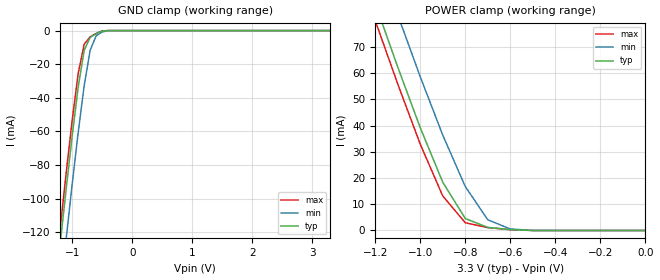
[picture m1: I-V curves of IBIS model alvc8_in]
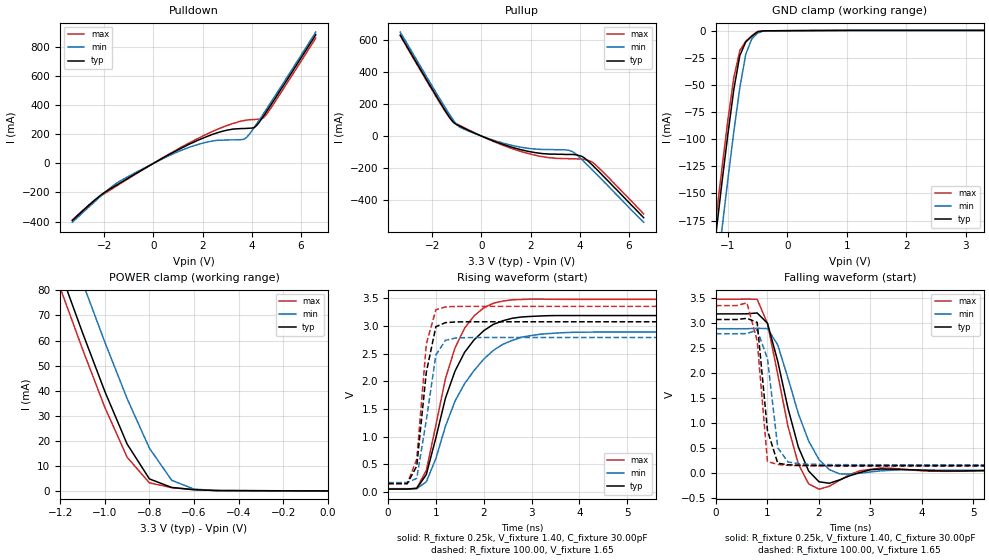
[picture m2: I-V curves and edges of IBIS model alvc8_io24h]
| IBIS file 32245ah.ibs created by s2ibis2 version 1.1
| North Carolina State University Electronics Research Laboratory  1995
[IBIS ver]   2.1
[File name]   32245ah.ibs
[File Rev]   1.0
[Date]   03/01/99
[Source]   Integrated Device Technology, Inc.
[Notes]   1.Temperatures: typ=25C, min=100C, max=0C 2.RRmp rates based
   on 50 ohm load.
[Disclaimer] Integrated Device Technology, Inc. ("IDT") hereby grants the
   user of this IBIS model a non-exclusive, nontransferable
   license to use this IBIS model under the following terms. The
   user is granted this license only to use the IBIS model and is
   not granted rights to sell, copy (except as needed to run the
   IBIS model), rent, lease or sub-license the IBIS model in
   whole or in part, or in modified form to anyone. The User may
   modify the IBIS model to suit its specific applications, but
   rights to derivative works and such modifications shall belong
   to IDT. This IBIS model is provided on an AS IS" basis and IDT
   makes absolutely no warranty with respect to the information
   contained herein. IDT DISCLAIMS AND CUSTOMER WAIVES ALL
   WARRANTIES, EXPRESS AND IMPLIED, INCLUDING WARRANTIES OF
   MERCHANTABILITY AND FITNESS FOR A PARTICULAR PURPOSE. THE
   ENTIRE RISK AS TO QUALITY AND PERFORMANCE IS WITH THE USER
   ACCORDINGLY, IN NO EVENT SHALL IDT BE LIABLE FOR ANY DIRECT OR
   INDIRECT DAMAGES, WHETHER IN CONTRACT OR TORT, INCLUDING ANY
   LOST PROFITS OR OTHER INCIDENTAL, CONSEQUENTIAL, EXEMPLARY, OR
   PUNITIVE DAMAGES ARISING OUT OF THE USE OR APPLICATION OF THE
   IBIS model. Further, IDT reserves the right to make changes
   without notice to any product herein to improve reliability,
   function, or design. IDT does not convey any license under
   patent rights or any other intellectual property rights,
   including those of third parties. IDT is not obligated to
   provide maintenance or support for the licensed IBIS model.
[Copyright]   Copyright 1997, Integrated Device Technology, Inc. all rights
   reserved
|   Component ALVCH32245
[Component]   ALVCH32245
[Manufacturer]   Integrated Device Technology
[Package]
| BF96
| variable   typ   min   max
R_pkg   144.3m   NA   NA
L_pkg   4.10nH   NA   NA
C_pkg   0.36pF   NA   NA
[Pin]  signal_name   model_name   R_pin   L_pin   C_pin
A1   1B2   alvc8_io24h
A2   1B1   alvc8_io24h
A3   1DIR   alvc8_in
A4   1OEB   alvc8_in
A5   1A1   alvc8_io24h
A6   1A2   alvc8_io24h
B1   1B4   alvc8_io24h
B2   1B3   alvc8_io24h
B3   GND   GND
B4   GND   GND
B5   1A3   alvc8_io24h
B6   1A4   alvc8_io24h
C1   1B6   alvc8_io24h
C2   1B5   alvc8_io24h
C3   VCC   POWER
C4   VCC   POWER
C5   1A5   alvc8_io24h
C6   1A6   alvc8_io24h
D1   1B8   alvc8_io24h
D2   1B7   alvc8_io24h
D3   GND   GND
D4   GND   GND
D5   1A7   alvc8_io24h
D6   1A8   alvc8_io24h
E1   2B2   alvc8_io24h
E2   2B1   alvc8_io24h
E3   GND   GND
E4   GND   GND
E5   2A1   alvc8_io24h
E6   2A2   alvc8_io24h
F1   2B4   alvc8_io24h
F2   2B3   alvc8_io24h
F3   VCC   POWER
F4   VCC   POWER
F5   2A3   alvc8_io24h
F6   2A4   alvc8_io24h
G1   2B6   alvc8_io24h
G2   2B5   alvc8_io24h
G3   GND   GND
G4   GND   GND
G5   2A5   alvc8_io24h
G6   2A6   alvc8_io24h
H1   2B7   alvc8_io24h
H2   2B8   alvc8_io24h
H3   2DIR   alvc8_in
H4   2OEB   alvc8_in
H5   2A8   alvc8_io24h
H6   2A7   alvc8_io24h
J1   3B2   alvc8_io24h
J2   3B1   alvc8_io24h
J3   3DIR   alvc8_in
J4   3OEB   alvc8_in
J5   3A1   alvc8_io24h
J6   3A2   alvc8_io24h
K1   3B4   alvc8_io24h
K2   3B3   alvc8_io24h
K3   GND   GND
K4   GND   GND
K5   3A3   alvc8_io24h
K6   3A4   alvc8_io24h
L1   3B6   alvc8_io24h
L2   3B5   alvc8_io24h
L3   VCC   POWER
L4   VCC   POWER
L5   3A5   alvc8_io24h
L6   3A6   alvc8_io24h
M1   3B8   alvc8_io24h
M2   3B7   alvc8_io24h
M3   GND   GND
M4   GND   GND
M5   3A7   alvc8_io24h
M6   3A8   alvc8_io24h
N1   4B2   alvc8_io24h
N2   4B1   alvc8_io24h
N3   GND   GND
N4   GND   GND
N5   4A1   alvc8_io24h
N6   4A2   alvc8_io24h
P1   4B4   alvc8_io24h
P2   4B3   alvc8_io24h
P3   VCC   POWER
P4   VCC   POWER
P5   4A3   alvc8_io24h
P6   4A4   alvc8_io24h
R1   4B6   alvc8_io24h
R2   4B5   alvc8_io24h
R3   GND   GND
R4   GND   GND
R5   4A5   alvc8_io24h
R6   4A6   alvc8_io24h
T1   4B7   alvc8_io24h
T2   4B8   alvc8_io24h
T3   4DIR   alvc8_in
T4   4OEB   alvc8_in
T5   4A8   alvc8_io24h
T6   4A7   alvc8_io24h
| Models and submodels in the file (2): alvc8_in (Input), alvc8_io24h (I/O)
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| in   in   dummy_model
| oe   oe   dummy_model
|   Model alvc8_in
[Model]   alvc8_in
Model_type   Input
Vinl =  0.800V
Vinh =  2.000V
C_comp   3.00pF   NA   NA
[Temperature Range]   25.00   100.00   0.000
[Voltage Range]   3.30V   3.00V   3.60V
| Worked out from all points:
|   GND clamp passes 1 mA (typ) near -0.54 V on its own axis
|   POWER clamp passes 1 mA (typ) near -0.68 V on its own axis
[GND_clamp]
| voltage   I(typ)   I(min)   I(max)
-3.3V     -860mA     -887mA     -851mA
-1.3V     -161mA     -190mA     -151mA
-1.2V     -127mA     -157mA     -118mA
-1.1V     -94.41mA   -124mA     -84.85mA
-1V       -62.78mA   -91.54mA   -53.52mA
-900mV    -33.71mA   -60.78mA   -25.6mA
-800mV    -11.74mA   -32.83mA   -8.09mA
-700mV    -4.033mA   -11.65mA   -3.7mA
-600mV    -1.899mA   -3.108mA   -1.699mA
-500mV    -308uA     -810uA     -172uA
-400mV    -3.848nA   -9.872uA   -399pA
3.3V      39.6pA     19.33nA    26.4pA
[POWER_clamp]
| voltage   I(typ)   I(min)   I(max)
-3.3V     630mA      648mA      624mA
-1.2V     86.56mA    106mA      80.02mA
-1.1V     62.33mA    82.22mA    55.88mA
-1V       39.2mA     58.61mA    32.91mA
-900mV    18.4mA     36.35mA    13.15mA
-800mV    4.556mA    16.76mA    2.954mA
-700mV    1.164mA    4.056mA    1.087mA
-600mV    320uA      578uA      299uA
-500mV    40.08nA    12.23uA    3.465nA
0V        39.6pA     59.11pA    43.2pA
|   Model alvc8_io24h
[Model]   alvc8_io24h
Model_type   I/O
Polarity   Non-Inverting
Enable   Active-High
Vinl =  0.000V
Vinh =  2.000V
Vmeas =  1.500V
C_comp   3.00pF   NA   NA
[Temperature Range]   25.00   100.00   0.000
[Voltage Range]   3.30V   3.00V   3.60V
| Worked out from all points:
|   slope of the pulldown table from 0 to 0.495 V, typ, clamps not added: 10.5 ohm
|   slope of the pullup table from 0 to 0.495 V, typ, clamps not added: 16.1 ohm
|   GND clamp passes 1 mA (typ) near -0.50 V on its own axis
|   POWER clamp passes 1 mA (typ) near -0.66 V on its own axis
|   rising waveform, R_fixture 0.25k, V_fixture 1.40, C_fixture 30.00pF: 20-80 % time 723ps typ, 920ps min, 623ps max; typ from 0.055 V to 3.19 V
|   rising waveform, R_fixture 100.00, V_fixture 1.65: 20-80 % time 248ps typ, 279ps min, 194ps max; typ from 0.155 V to 3.08 V
|   falling waveform, R_fixture 0.25k, V_fixture 1.40, C_fixture 30.00pF: 20-80 % time 444ps typ, 538ps min, 413ps max; typ from 3.19 V to 0.055 V
|   falling waveform, R_fixture 100.00, V_fixture 1.65: 20-80 % time 187ps typ, 176ps min, 171ps max; typ from 3.08 V to 0.155 V
[Pulldown]
| voltage   I(typ)   I(min)   I(max)
-3.3V     -392mA     -404mA     -389mA
-2.3V     -240mA     -249mA     -241mA
-1.5V     -149mA     -136mA     -156mA
300mV     28.8mA     25.5mA     30.3mA
1.4V      127mA      107mA      135mA
2.4V      199mA      153mA      219mA
3.6V      239mA      163mA      291mA
3.8V      240mA      180mA      297mA
4.2V      260mA      272mA      302mA
4.4V      306mA      322mA      306mA
4.6V      356mA      373mA      337mA
6.6V      883mA      901mA      860mA
[Pullup]
| voltage   I(typ)   I(min)   I(max)
-3.3V     630mA      649mA      628mA
-1.4V     142mA      160mA      137mA
-1.1V     80.6mA     90.7mA     83.6mA
-900mV    63mA       57.7mA     67.6mA
400mV     -25.1mA    -21.5mA    -27.4mA
1.6V      -85mA      -69.5mA    -95.9mA
2.6V      -111mA     -84mA      -132mA
3.4V      -115mA     -86.1mA    -141mA
3.7V      -115mA     -97.1mA    -142mA
4.1V      -128mA     -149mA     -144mA
4.5V      -179mA     -210mA     -162mA
6.6V      -510mA     -538mA     -486mA
[GND_clamp]
| voltage   I(typ)   I(min)   I(max)
-3.3V     -1.238A    -1.278A    -1.225A
-1.3V     -235mA     -278mA     -221mA
-1.2V     -187mA     -230mA     -173mA
-1.1V     -140mA     -183mA     -127mA
-1V       -95.39mA   -137mA     -82.2mA
-900mV    -54.08mA   -92.95mA   -42.96mA
-800mV    -22.96mA   -52.74mA   -18.28mA
-700mV    -10.43mA   -21.77mA   -9.816mA
-600mV    -5.251mA   -7.746mA   -4.745mA
-500mV    -1.015mA   -2.281mA   -688uA
-400mV    -144uA     -128uA     -169uA
3.3V      264uA      161uA      341uA
[POWER_clamp]
| voltage   I(typ)   I(min)   I(max)
-3.3V     638mA      656mA      632mA
-1.2V     87.67mA    108mA      81.05mA
-1.1V     63.19mA    83.28mA    56.62mA
-1V       39.75mA    59.43mA    33.41mA
-900mV    18.73mA    36.86mA    13.47mA
-800mV    4.8mA      17.05mA    3.222mA
-700mV    1.374mA    4.243mA    1.32mA
-600mV    498uA      728uA      497uA
-500mV    146uA      134uA      162uA
0V        111pA      156pA      121pA
[Ramp]
| variable   typ   min   max
dV/dt_r   1.48/0.31n   1.29/0.30n   1.66/0.22n
dV/dt_f   1.63/0.28n   1.45/0.31n   1.80/0.19n
R_load = 50.00
[Rising Waveform]
R_fixture = 0.25k
V_fixture = 1.40
C_fixture = 30.00pF
R_dut = 7.00m
L_dut = 3.30nH
C_dut = 0.29pF
| time   V(typ)   V(min)   V(max)
0s        55.43mV    62mV       53.03mV
600ps     66.6mV     63.52mV    70.73mV
800ps     318mV      185mV      393mV
1ns       982mV      608mV      1.211V
1.2ns     1.697V     1.189V     2.05V
1.4ns     2.186V     1.644V     2.606V
1.8ns     2.751V     2.198V     3.185V
2.4ns     3.095V     2.67V      3.451V
3.8ns     3.189V     2.885V     3.481V
19.8ns    3.189V     2.893V     3.482V
[Rising Waveform]
R_fixture = 100.00
V_fixture = 1.65
R_dut = 7.00m
L_dut = 3.30nH
C_dut = 0.29pF
| time   V(typ)   V(min)   V(max)
0s        155mV      172mV      148mV
400ps     155mV      173mV      148mV
600ps     469mV      249mV      594mV
800ps     2.166V     1.299V     2.675V
1ns       2.988V     2.477V     3.294V
1.2ns     3.061V     2.741V     3.346V
1.4ns     3.073V     2.782V     3.353V
2ns       3.077V     2.793V     3.355V
19.8ns    3.077V     2.793V     3.355V
[Falling Waveform]
R_fixture = 0.25k
V_fixture = 1.40
C_fixture = 30.00pF
R_dut = 7.00m
L_dut = 3.30nH
C_dut = 0.29pF
| time   V(typ)   V(min)   V(max)
0s        3.189V     2.893V     3.482V
800ps     3.208V     2.901V     3.481V
1ns       3.002V     2.896V     2.998V
1.2ns     2.239V     2.568V     1.977V
1.4ns     1.294V     1.899V     934mV
1.6ns     525mV      1.193V     186mV
2ns       -168mV     277mV      -316mV
2.4ns     -131mV     -10.2mV    -138mV
3.2ns     86.4mV     50.55mV    107mV
19.8ns    55.43mV    62mV       53.03mV
[Falling Waveform]
R_fixture = 100.00
V_fixture = 1.65
R_dut = 7.00m
L_dut = 3.30nH
C_dut = 0.29pF
| time   V(typ)   V(min)   V(max)
0s        3.077V     2.793V     3.355V
400ps     3.077V     2.793V     3.355V
600ps     3.101V     2.795V     3.411V
800ps     3.02V      2.869V     2.651V
1ns       857mV      2.294V     237mV
1.2ns     202mV      512mV      177mV
1.4ns     172mV      227mV      160mV
1.6ns     163mV      194mV      154mV
2ns       157mV      178mV      149mV
19.8ns    155mV      172mV      148mV
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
